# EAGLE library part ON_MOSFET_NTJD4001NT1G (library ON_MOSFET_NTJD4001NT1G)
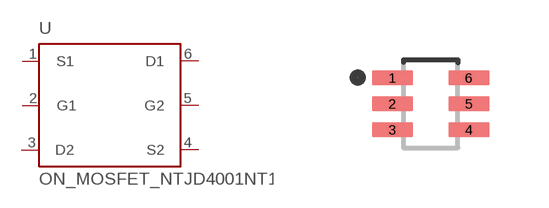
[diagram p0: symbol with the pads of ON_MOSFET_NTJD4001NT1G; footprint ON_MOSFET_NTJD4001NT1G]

Designator prefix -

## ON_MOSFET_NTJD4001NT1GRPI  [ON_MOSFET_NTJD4001NT1G]
1  S1  out
2  G1  in
3  D2  in
4  S2  out
5  G2  in
6  D1  in

## Footprint ON_MOSFET_NTJD4001NT1G (pad centres in mm)
smd 1.02 x 0.36: 1 -0.955,0.65; 2 -0.955,0; 3 -0.955,-0.65; 4 0.955,-0.65; 5 0.955,0; 6 0.955,0.65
